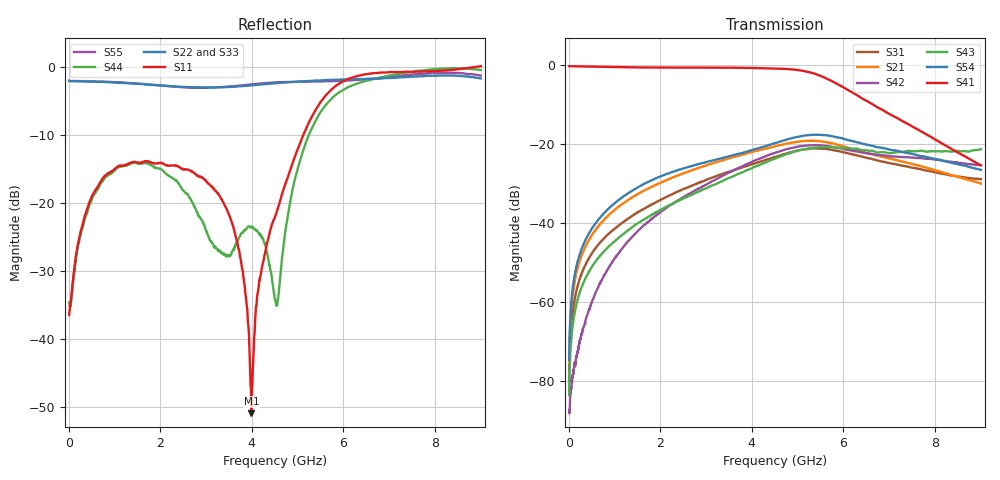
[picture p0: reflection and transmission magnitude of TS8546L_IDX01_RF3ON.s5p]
# GHz S DB R 50
! CMT, SN0916, 25263762, 26.7.0
! Date: 16.07.2026 12:22:49
! Data: Format
! Freq S1.1:dB/Ang S1.2:dB/Ang S1.3:dB/Ang S1.4:dB/Ang S1.5:dB/Ang
!  S2.1:dB/Ang S2.2:dB/Ang S2.3:dB/Ang S2.4:dB/Ang S2.5:dB/Ang
!  S3.1:dB/Ang S3.2:dB/Ang S3.3:dB/Ang S3.4:dB/Ang S3.5:dB/Ang
!  S4.1:dB/Ang S4.2:dB/Ang S4.3:dB/Ang S4.4:dB/Ang S4.5:dB/Ang
!  S5.1:dB/Ang S5.2:dB/Ang S5.3:dB/Ang S5.4:dB/Ang S5.5:dB/Ang
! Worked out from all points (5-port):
!   2001 points, 10 MHz to 9 GHz, reference 50 ohm
!   strongest paths, dB at 10 MHz, 2.257 GHz, 4.505 GHz, 6.753 GHz, 9 GHz:
!     S41: -0.2, -0.5, -0.8, -10.7, -25.3
!     S54: -74.7, -27.1, -19.7, -20.8, -26.5
!     S43: -83.6, -35.2, -23.7, -22.1, -21.3
!     S42: -87.6, -35.2, -22.2, -22.7, -25.3
!     S21: -75.4, -28.5, -20.5, -22.9, -30.0
!     S31: -80.0, -32.7, -23.2, -24.1, -28.9
!   lowest |S11| = -50.9 dB at 3.988 GHz (marker M1), VSWR 1.01, Z = 49.8 + j0.15 ohm
!   |S11| at or under -10 dB: start of sweep to 5.126 GHz
